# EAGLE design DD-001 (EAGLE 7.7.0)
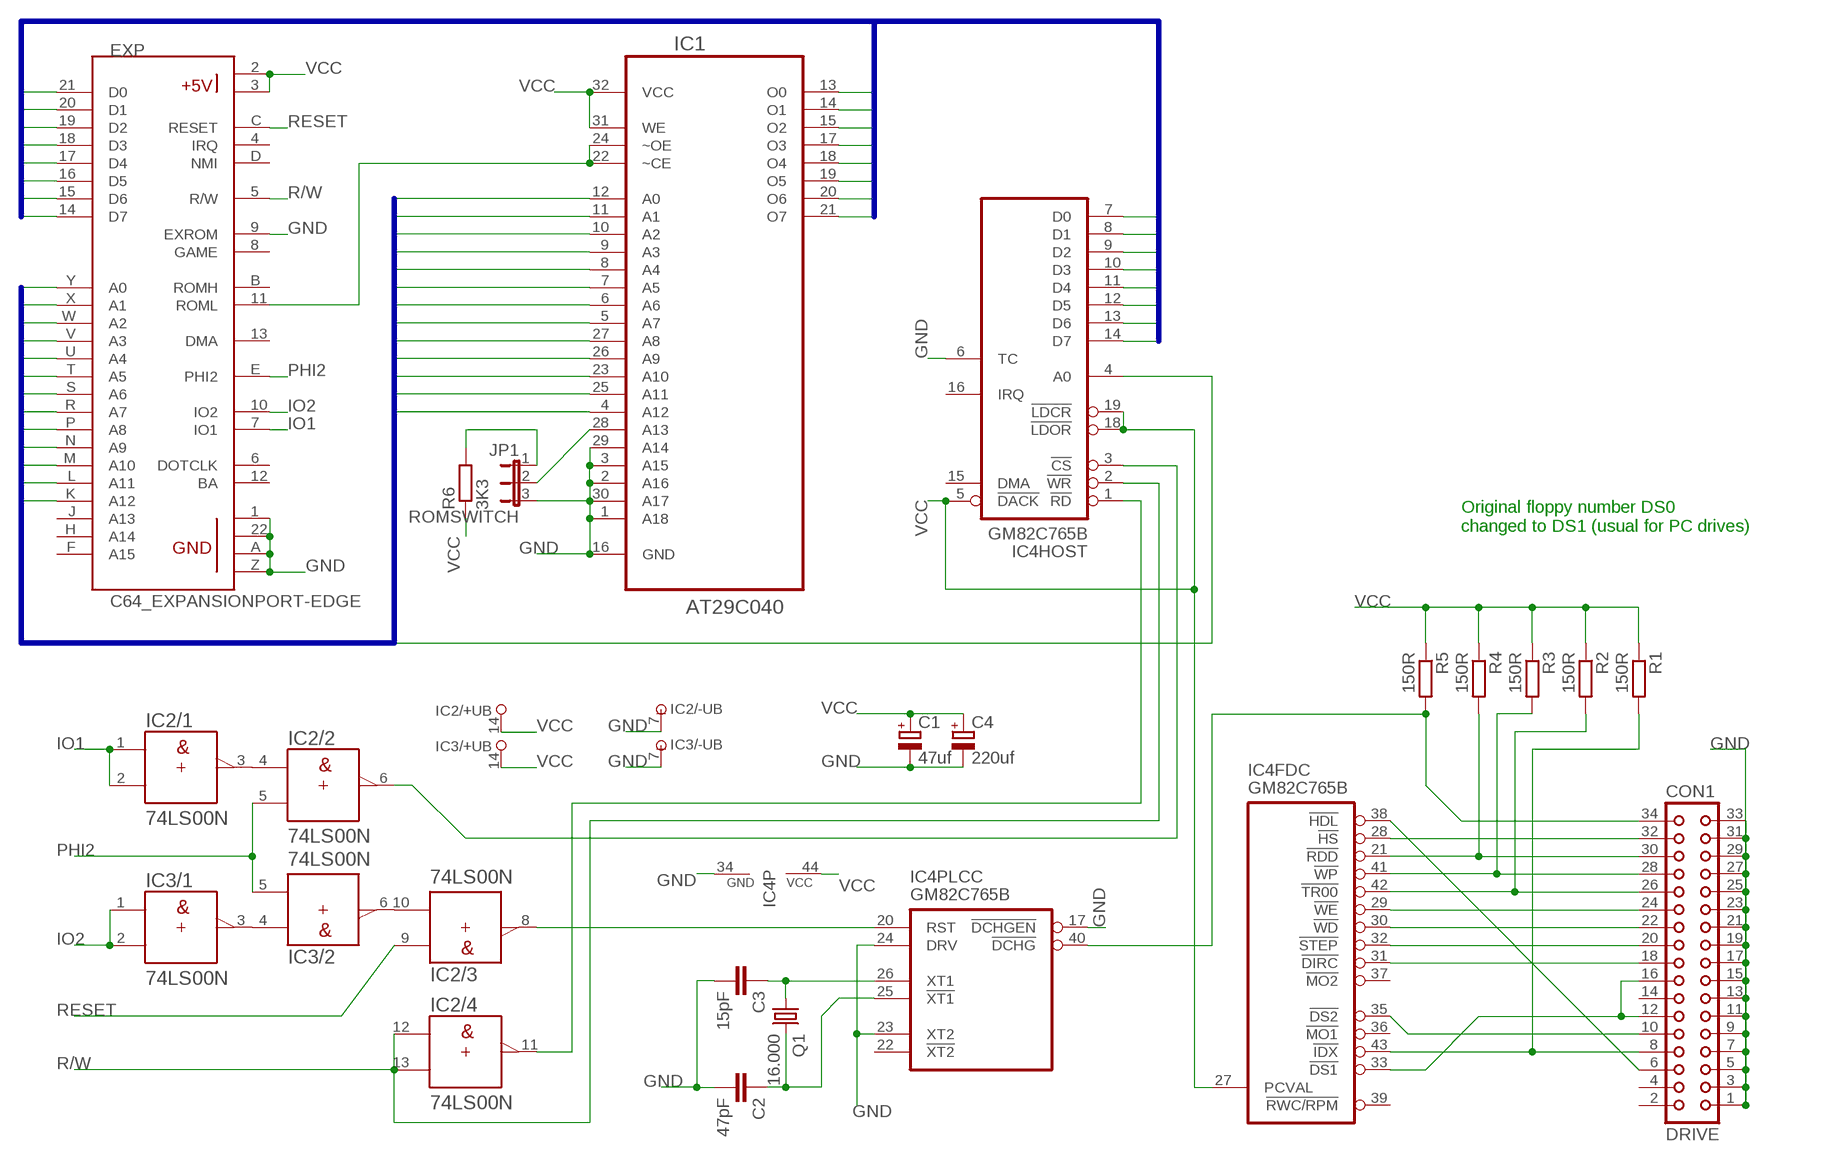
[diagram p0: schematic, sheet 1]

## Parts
C1  47uf  CPOL-EUE2.5-5  [E2,5-5]
C2  47pF  C-EU050-024X044  [C050-024X044]
C3  15pF  C-EU050-024X044  [C050-024X044]
C4  220uf  CPOL-EUE5-6  [E5-6]
CON1  DRIVE  CON34L  [CON34L]
EXP  C64_EXPANSIONPORT-EDGE  [EXPANSIONPORT-C64-EDGE]
IC1  AT29C040  [DIP254P1524X482-32]
IC2  74LS00N  [DIL14]
IC3  74LS00N  [DIL14]
IC4  GM82C765B  3765_PLCC  [PLCC44]
JP1  ROMSWITCH  JP2W  [JP2W]
Q1  16.000  CRYSTALHC49S  [HC49/S]
R1  150R  R-EU_0207/10  [0207/10]
R2  150R  R-EU_0207/10  [0207/10]
R3  150R  R-EU_0207/10  [0207/10]
R4  150R  R-EU_0207/10  [0207/10]
R5  150R  R-EU_0207/10  [0207/10]
R6  3K3  R-EU_R1206  [R1206]

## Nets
_XT1: C2.1 IC4.25(PLCC:!XT1) Q1.2
A0: EXP.Y(A0) IC1.12(A0) IC4.4(HOST:A0)
A1: EXP.X(A1) IC1.11(A1)
A2: EXP.W(A2) IC1.10(A2)
A3: EXP.V(A3) IC1.9(A3)
A4: EXP.U(A4) IC1.8(A4)
A5: EXP.T(A5) IC1.7(A5)
A6: EXP.S(A6) IC1.6(A6)
A7: EXP.R(A7) IC1.5(A7)
A8: EXP.P(A8) IC1.27(A8)
A9: EXP.N(A9) IC1.26(A9)
A10: EXP.M(A10) IC1.23(A10)
A11: EXP.L(A11) IC1.25(A11)
A12: EXP.K(A12) IC1.4(A12)
A13: IC1.28(A13) JP1.2
CS: IC2.6(/2:Y) IC4.3(HOST:!CS)
D0: EXP.21(D0) IC1.13(O0) IC4.7(HOST:D0)
D1: EXP.20(D1) IC1.14(O1) IC4.8(HOST:D1)
D2: EXP.19(D2) IC1.15(O2) IC4.9(HOST:D2)
D3: EXP.18(D3) IC1.17(O3) IC4.10(HOST:D3)
D4: EXP.17(D4) IC1.18(O4) IC4.11(HOST:D4)
D5: EXP.16(D5) IC1.19(O5) IC4.12(HOST:D5)
D6: EXP.15(D6) IC1.20(O6) IC4.13(HOST:D6)
D7: EXP.14(D7) IC1.21(O7) IC4.14(HOST:D7)
DCHG: CON1.34 IC4.40(PLCC:!DCHG) R5.2
DIR: CON1.18 IC4.31(FDC:!DIRC)
DS1: CON1.12 CON1.16 IC4.33(FDC:!DS1)
DS2: CON1.10 IC4.35(FDC:!DS2)
GND: C1.- C2.2 C3.2 C4.- CON1.1 CON1.3 CON1.5 CON1.7 CON1.9 CON1.11 CON1.13 CON1.15 CON1.17 CON1.19 CON1.21 CON1.23 CON1.25 CON1.27 CON1.29 CON1.31 CON1.33 EXP.1(GND1) EXP.9(EXROM) EXP.22(GND2) EXP.A(GND3) EXP.Z(GND4) IC1.1(A18) IC1.2(A16) IC1.3(A15) IC1.16(GND) IC1.29(A14) IC1.30(A17) IC2.7(/-UB:-UB) IC3.7(/-UB:-UB) IC4.6(HOST:TC) IC4.17(PLCC:!DCHGEN) IC4.23(PLCC:XT2) IC4.24(PLCC:DRV) IC4.34(P:GND) JP1.3
HDL: CON1.6 IC4.38(FDC:!HDL)
HI_ROM: JP1.1 R6.2
HS: CON1.32 IC4.28(FDC:!HS)
IDX: CON1.8 IC4.43(FDC:!IDX) R1.2
IO1: EXP.7(IO1) IC2.1(/1:A) IC2.2(/1:B)
IO1N: IC2.3(/1:Y) IC2.4(/2:A)
IO2: EXP.10(IO2) IC3.1(/1:A) IC3.2(/1:B)
IO2N: IC3.3(/1:Y) IC3.4(/2:A)
IO2RES: IC2.10(/3:B) IC3.6(/2:Y)
PHI2: EXP.E(PHI2) IC2.5(/2:B) IC3.5(/2:B)
R/W: EXP.5(R/W) IC2.12(/4:A) IC2.13(/4:B) IC4.2(HOST:!WR)
RD: IC2.11(/4:Y) IC4.1(HOST:!RD)
RDD: CON1.30 IC4.21(FDC:!RDD) R4.2
RESET: EXP.C(RESET) IC2.9(/3:A)
ROML: EXP.11(ROML) IC1.22(~CE) IC1.24(~OE)
RST: IC2.8(/3:Y) IC4.20(PLCC:RST)
STEP: CON1.20 IC4.32(FDC:!STEP)
TR00: CON1.26 IC4.42(FDC:!TR00) R2.2
VCC: C1.+ C4.+ EXP.2(+5V1) EXP.3(+5V2) IC1.31(WE) IC1.32(VCC) IC2.14(/+UB:+UB) IC3.14(/+UB:+UB) IC4.5(HOST:!DACK) IC4.18(HOST:!LDOR) IC4.19(HOST:!LDCR) IC4.27(FDC:PCVAL) IC4.44(P:VCC) R1.1 R2.1 R3.1 R4.1 R5.1 R6.1
WD: CON1.22 IC4.30(FDC:!WD)
WE: CON1.24 IC4.29(FDC:!WE)
WP: CON1.28 IC4.41(FDC:!WP) R3.2
XT1: C3.1 IC4.26(PLCC:XT1) Q1.1
Unconnected: CON1.2 CON1.4 CON1.14 EXP.4(IRQ) EXP.6(DOTCLK) EXP.8(GAME) EXP.12(BA) EXP.13(DMA) EXP.B(ROMH) EXP.D(NMI) EXP.F(A15) EXP.H(A14) EXP.J(A13) IC3.8(/3:Y) IC3.9(/3:A) IC3.10(/3:B) IC3.11(/4:Y) IC3.12(/4:A) IC3.13(/4:B) IC4.15(HOST:DMA) IC4.16(HOST:IRQ) IC4.22(PLCC:!XT2) IC4.36(FDC:!MO1) IC4.37(FDC:!MO2) IC4.39(FDC:!RWC/RPM)

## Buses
D[0..7]
A[0..12]

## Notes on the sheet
- Original floppy number DS0
  changed to DS1 (usual for PC drives)

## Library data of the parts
C1 C4 = resistor:CPOL-EU: POLARIZED CAPACITOR, European symbol
C2 C3 = rcl:C-EU: CAPACITOR, European symbol
CON1 = con-harting:CON34L: CONNECTOR; OC_FARNELL: unknown; OC_NEWARK: unknown
EXP = commodore:C64_EXPANSIONPORT-EDGE: expansion port for the Commodore 64, edge/cartridge version
IC1 = Atmel_By_element14_Batch_1-00:AT29C040: 4-Megabit (512K x 8) OTP EPROM; MPN: AT29C040; OC_FARNELL: 1455024; OC_NEWARK: 58M3822; PACKAGE: PDIP-32; SUPPLIER: Atmel
IC2 IC3 = 74ttl-din:74*00: Quad 2-input NAND gate
IC4 = oldchips3:3765_PLCC: 3765 PLCC Floppy Disk Controller
JP1 = jumper:JP2W: JUMPER
Q1 = crystal:CRYSTAL: CRYSTAL; OC_FARNELL: 1667008; OC_NEWARK: unknown
R1-R6 = resistor:R-EU_: RESISTOR, European symbol

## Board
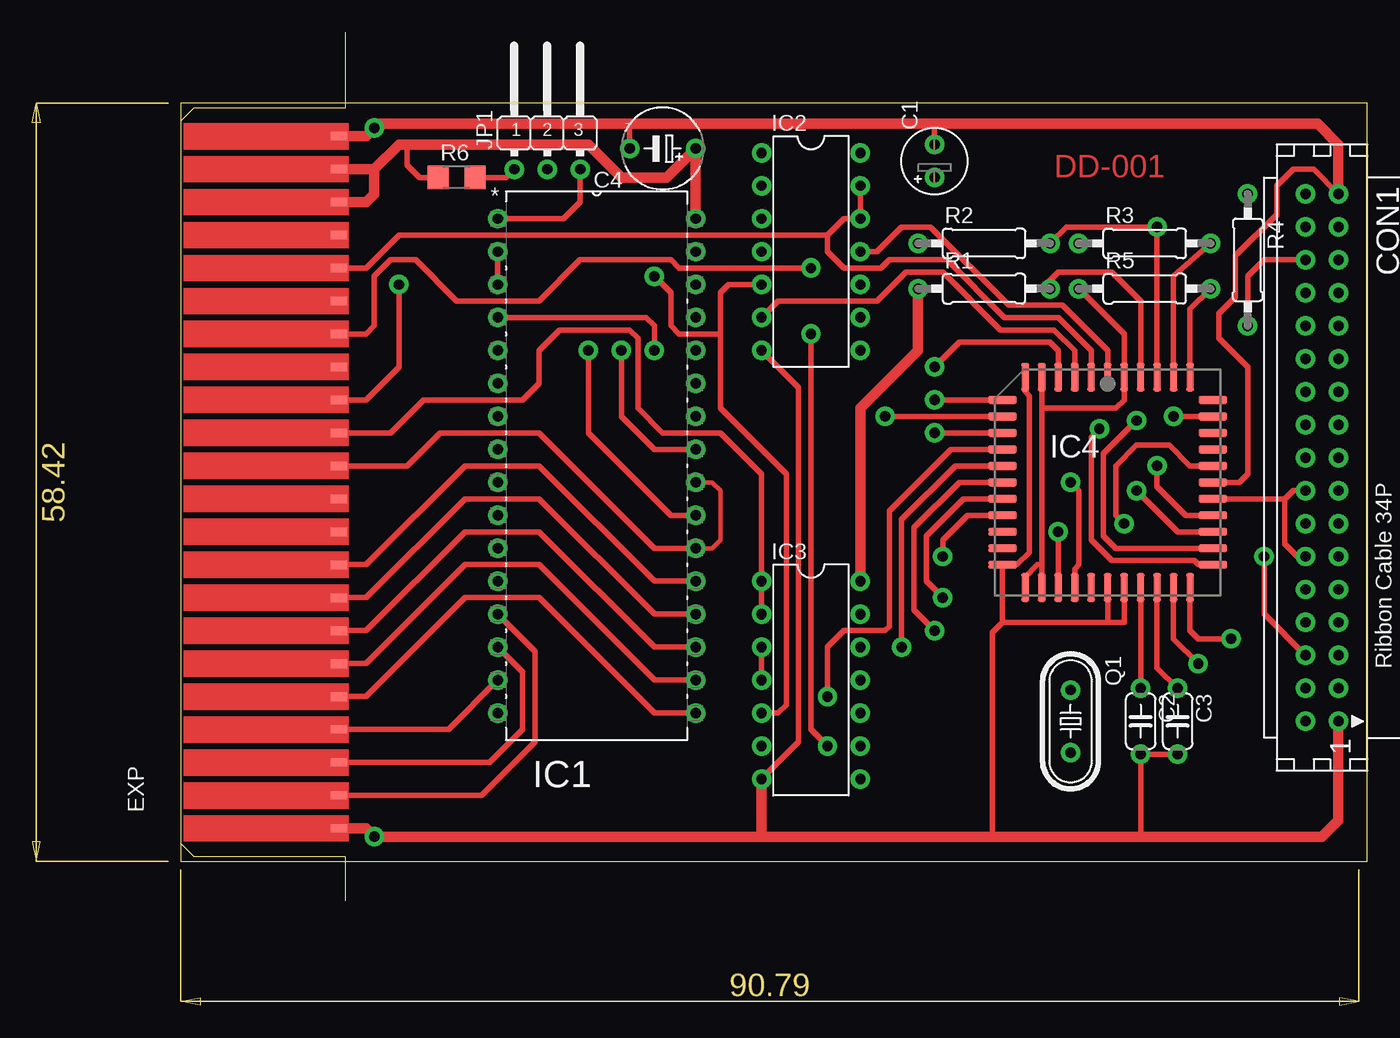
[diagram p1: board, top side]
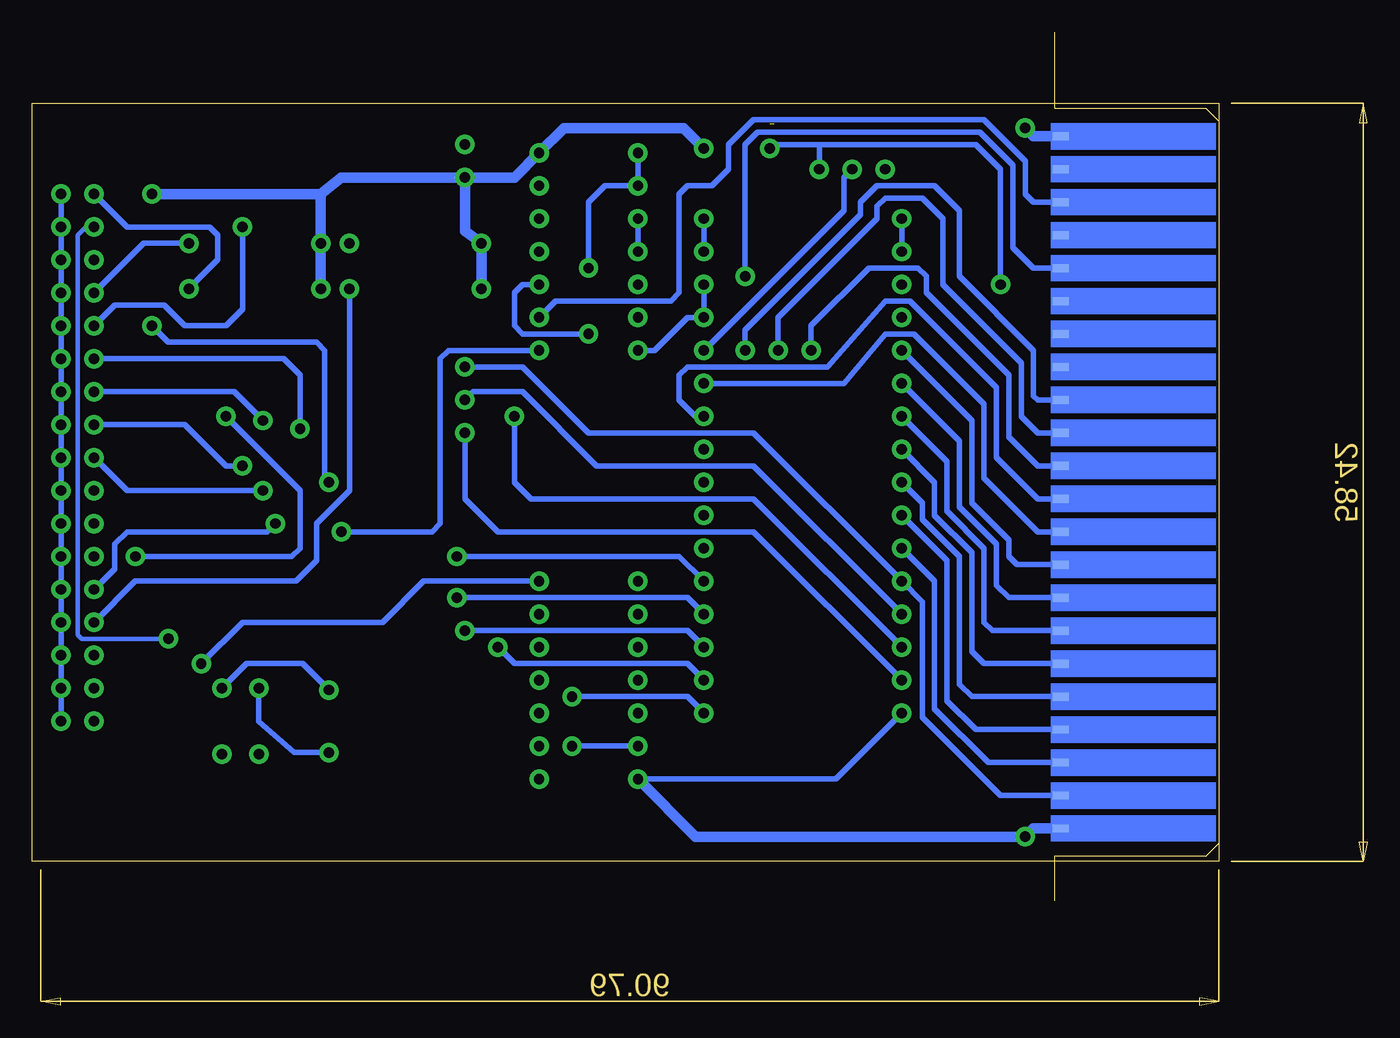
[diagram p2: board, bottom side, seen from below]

Size 102.84 x 74.98 mm. Coordinates in mm from the lower left corner, seen from the top.
Outline: 11.41,11.1 102.84,11.1 102.84,69.5 11.41,69.5 11.41,11.1
Copper layers (1*16): Top 0.035mm / dielectric 1.5mm / Bottom 0.035mm
Design rules "default *": minimum track width 10mil, minimum drill 24mil, track to track 10mil, track to pad 10mil, pad to pad 10mil, via to via 10mil, smd to smd 10mil, copper to edge 40mil, drill to drill 8mil, minimum pad ring 10mil, minimum via ring 8mil, stop-mask expansion 4mil, vias tented up to drill 0mil, thermal gap 10mil

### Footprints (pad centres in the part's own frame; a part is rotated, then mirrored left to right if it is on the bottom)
E2,5-5 = drill 0.8 pad 1.499: + -1.27,0; - 1.27,0
C050-024X044 = drill 0.8 pad 1.499: 1 -2.54,0; 2 2.54,0
E5-6 = drill 0.8 pad 1.499: + -2.54,0; - 2.54,0
CON34L = drill 0.8 pad 1.499: 1 20.32,1.27; 2 20.32,-1.27; 3 17.78,1.27; 4 17.78,-1.27; 5 15.24,1.27; 6 15.24,-1.27; 7 12.7,1.27; 8 12.7,-1.27; 9 10.16,1.27; 10 10.16,-1.27; 11 7.62,1.27; 12 7.62,-1.27; 13 5.08,1.27; 14 5.08,-1.27; 15 2.54,1.27; 16 2.54,-1.27; 17 0,1.27; 18 0,-1.27; 19 -2.54,1.27; 20 -2.54,-1.27; 21 -5.08,1.27; 22 -5.08,-1.27; 23 -7.62,1.27; 24 -7.62,-1.27; 25 -10.16,1.27; 26 -10.16,-1.27; 27 -12.7,1.27; 28 -12.7,-1.27; 29 -15.24,1.27; 30 -15.24,-1.27; 31 -17.78,1.27; 32 -17.78,-1.27; 33 -20.32,1.27; 34 -20.32,-1.27
EXPANSIONPORT-C64-EDGE = smd 0.635 x 1.27: 1 2.54,12.192; 2 5.08,12.192; 3 7.62,12.192; 4 10.16,12.192; 5 12.7,12.192; 6 15.24,12.192; 7 17.78,12.192; 8 20.32,12.192; 9 22.86,12.192; 10 25.4,12.192; 11 27.94,12.192; 12 30.48,12.192; 13 33.02,12.192; 14 35.56,12.192; 15 38.1,12.192; 16 40.64,12.192; 17 43.18,12.192; 18 45.72,12.192; 19 48.26,12.192; 20 50.8,12.192; 21 53.34,12.192; 22 55.88,12.192 | smd 0.635 x 1.27 bottom: A 2.54,12.192; B 5.08,12.192; C 7.62,12.192; D 10.16,12.192; E 12.7,12.192; F 15.24,12.192; H 17.78,12.192; J 20.32,12.192; K 22.86,12.192; L 25.4,12.192; M 27.94,12.192; N 30.48,12.192; P 33.02,12.192; R 35.56,12.192; S 38.1,12.192; T 40.64,12.192; U 43.18,12.192; V 45.72,12.192; W 48.26,12.192; X 50.8,12.192; Y 53.34,12.192; Z 55.88,12.192
DIP254P1524X482-32 = drill 0.8 pad 1.499: 1 -15.24,38.1; 2 -15.24,35.56; 3 -15.24,33.02; 4 -15.24,30.48; 5 -15.24,27.94; 6 -15.24,25.4; 7 -15.24,22.86; 8 -15.24,20.32; 9 -15.24,17.78; 10 -15.24,15.24; 11 -15.24,12.7; 12 -15.24,10.16; 13 -15.24,7.62; 14 -15.24,5.08; 15 -15.24,2.54; 16 -15.24,0; 17 0,0; 18 0,2.54; 19 0,5.08; 20 0,7.62; 21 0,10.16; 22 0,12.7; 23 0,15.24; 24 0,17.78; 25 0,20.32; 26 0,22.86; 27 0,25.4; 28 0,27.94; 29 0,30.48; 30 0,33.02; 31 0,35.56; 32 0,38.1
DIL14 = drill 0.8 pad 1.499: 1 -7.62,-3.81; 2 -5.08,-3.81; 3 -2.54,-3.81; 4 0,-3.81; 5 2.54,-3.81; 6 5.08,-3.81; 7 7.62,-3.81; 8 7.62,3.81; 9 5.08,3.81; 10 2.54,3.81; 11 0,3.81; 12 -2.54,3.81; 13 -5.08,3.81; 14 -7.62,3.81
PLCC44 = smd 0.6 x 2.2: 1 0,6.83; 2 -1.27,6.83; 3 -2.54,6.83; 4 -3.81,6.83; 5 -5.08,6.83; 6 -6.35,6.83; 18 -6.35,-9.37; 19 -5.08,-9.37; 20 -3.81,-9.37; 21 -2.54,-9.37; 22 -1.27,-9.37; 23 0,-9.37; 24 1.27,-9.37; 25 2.54,-9.37; 26 3.81,-9.37; 27 5.08,-9.37; 28 6.35,-9.37; 40 6.35,6.83; 41 5.08,6.83; 42 3.81,6.83; 43 2.54,6.83; 44 1.27,6.83 | smd 2.2 x 0.6: 7 -8.1,5.08; 8 -8.1,3.81; 9 -8.1,2.54; 10 -8.1,1.27; 11 -8.1,0; 12 -8.1,-1.27; 13 -8.1,-2.54; 14 -8.1,-3.81; 15 -8.1,-5.08; 16 -8.1,-6.35; 17 -8.1,-7.62; 29 8.1,-7.62; 30 8.1,-6.35; 31 8.1,-5.08; 32 8.1,-3.81; 33 8.1,-2.54; 34 8.1,-1.27; 35 8.1,0; 36 8.1,1.27; 37 8.1,2.54; 38 8.1,3.81; 39 8.1,5.08
JP2W = drill 0.8 pad 1.499: 1 -2.54,-1.27; 2 0,-1.27; 3 2.54,-1.27
HC49/S = drill 0.8 pad 1.499: 1 -2.413,0; 2 2.413,0
0207/10 = drill 0.8 pad 1.499: 1 -5.08,0; 2 5.08,0
R1206 = smd 1.6 x 1.803: 1 -1.422,0; 2 1.422,0

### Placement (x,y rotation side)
C1  69.52,65.07 90 top
C2  85.39,21.89 270 top
C3  88.25,21.89 270 top
C4  48.56,66.02 180 top
CON1  99.36,42.21 270 top
EXP  11.41,69.52 270 top
IC1  51.1,22.53 0 top
IC2  59.99,58.08 270 top
IC3  59.99,25.07 270 top
IC4  82.85,41.57 0 top
JP1  39.67,65.7 0 top
Q1  79.99,21.89 270 top
R1  73.33,55.23 0 top
R2  73.33,58.72 0 top
R3  85.71,58.72 0 top
R4  93.64,57.45 270 top
R5  85.71,55.23 0 top
R6  32.69,63.8 0 top

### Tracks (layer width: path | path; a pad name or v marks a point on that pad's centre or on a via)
_XT1
  Top 0.406: C2.1 IC4.25
  Bottom 0.406: Q1.2 82.66,19.48 85.39,21.89 C2.1
A0  (via drill 0.8 pad 1.5)
  Top 0.406: v69.52,49.2 71.42,51.1 78.41,51.1 79.04,50.46 IC4.4
  Bottom 0.406: v69.52,49.2 65.07,49.2 59.99,44.11 47.29,44.11 IC1.12 34.27,31.1 34.27,22.21 28.24,16.18 EXP.Y
A1
  Bottom 0.406: IC1.11 33.32,32.68 33.32,22.84 29.19,18.71 EXP.X
A2
  Bottom 0.406: IC1.10 32.37,34.27 32.37,23.48 30.15,21.26 EXP.W
A3
  Bottom 0.406: IC1.9 34.27,38.72 34.27,37.45 31.41,34.59 31.41,24.75 30.46,23.8 EXP.V
A4
  Bottom 0.406: IC1.8 33.32,40.3 33.32,37.77 30.46,34.91 30.46,27.29 29.51,26.34 EXP.U
A5
  Bottom 0.406: IC1.7 32.37,41.89 32.37,38.08 29.51,35.22 29.51,29.51 28.88,28.88 EXP.T
A6
  Bottom 0.406: IC1.6 31.41,43.48 31.41,38.4 28.56,35.54 28.56,32.37 27.61,31.42 EXP.S
A7
  Bottom 0.406: IC1.5 30.46,45.07 30.46,38.72 27.61,35.86 27.61,34.59 26.97,33.95 EXP.R
A8
  Bottom 0.406: IC1.27 40.3,47.92 37.13,51.73 34.91,51.73 29.51,46.34 29.51,40.62 25.38,36.49 EXP.P
A9
  Bottom 0.406: IC1.26 51.73,45.38 53.01,46.66 53.01,48.56 52.37,49.2 41.58,49.2 37.13,54.27 35.23,54.27 28.56,47.61 28.56,42.21 25.38,39.03 EXP.N 23.8,39.03
A10  (via drill 0.8 pad 1.5)
  Top 0.406: v42.85,50.46 42.85,44.11 49.2,37.77 IC1.23
  Bottom 0.406: v42.85,50.46 42.85,52.37 38.4,56.81 34.59,56.81 33.95,56.18 33.95,54.91 27.61,48.56 27.61,43.8 25.38,41.57 EXP.M
A11  (via drill 0.8 pad 1.5)
  Top 0.406: v45.39,50.46 45.39,45.38 47.93,42.84 IC1.25
  Bottom 0.406: v45.39,50.46 45.39,53 37.77,60.62 37.77,61.58 37.13,62.21 34.27,62.21 32.69,60.62 32.69,55.54 26.65,49.51 26.65,45.38 25.38,44.11 EXP.L
A12  (via drill 0.8 pad 1.5)
  Top 0.406: IC1.4 47.29,53 47.93,52.37 v47.93,50.46
  Bottom 0.406: v47.93,50.46 47.93,52.05 39.04,60.94 39.04,61.89 37.77,63.16 33.32,63.16 31.41,61.26 31.41,56.18 25.7,50.46 25.7,46.97 25.38,46.66 EXP.K
A13
  Bottom 0.406: IC1.28 40.3,61.26 40.3,63.8 JP1.2
CS
  Top 0.406: IC4.3 80.31,50.46 78.72,52.05 74.59,52.05 70.15,56.5 67.29,56.5 65.07,54.27 57.45,54.27 IC2.6
D0  (via drill 0.8 pad 1.5)
  Top 0.406: IC1.13 38.72,27.29 38.72,20.3 34.59,16.18 EXP.21 | IC4.7 v69.52,46.66
  Bottom 0.406: v69.52,46.66 68.88,47.29 65.07,47.29 59.36,41.57 47.29,41.57 IC1.13
D1  (via drill 0.8 pad 1.5)
  Top 0.406: IC1.14 37.77,25.7 37.77,21.26 35.23,18.71 EXP.20 | IC4.8 v65.7,45.38
  Bottom 0.406: IC1.14 47.29,39.03 64.44,39.03 65.7,40.3 v65.7,45.38
D2  (via drill 0.8 pad 1.5)
  Top 0.406: IC1.15 32.05,21.26 EXP.19 23.8,21.26 | IC4.9 v69.52,44.11
  Bottom 0.406: IC1.15 47.29,36.49 66.97,36.49 69.52,39.03 v69.52,44.11
D3  (via drill 0.8 pad 1.5)
  Top 0.406: EXP.18 25.7,23.8 33.32,31.42 39.04,31.42 47.93,22.53 IC1.17 | v61.26,23.8 61.26,27.61 62.53,28.88 65.7,28.88 66.02,29.19 66.02,38.08 70.78,42.84 IC4.10
  Bottom 0.406: v61.26,23.8 52.37,23.8 IC1.17
D4  (via drill 0.8 pad 1.5)
  Top 0.406: EXP.17 25.7,26.34 33.32,33.95 39.04,33.95 47.93,25.07 IC1.18 | v66.97,27.61 66.97,37.45 71.1,41.57 IC4.11
  Bottom 0.406: v66.97,27.61 65.7,26.34 52.37,26.34 IC1.18
D5  (via drill 0.8 pad 1.5)
  Top 0.406: EXP.16 25.7,28.88 33.32,36.49 39.04,36.49 47.93,27.61 IC1.19 | v69.52,28.88 67.93,30.46 67.93,36.81 71.42,40.3 IC4.12
  Bottom 0.406: v69.52,28.88 52.37,28.88 IC1.19
D6  (via drill 0.8 pad 1.5)
  Top 0.406: EXP.15 25.7,31.42 33.32,39.03 39.04,39.03 47.93,30.14 IC1.20 | v70.15,31.42 68.88,32.68 68.88,36.18 71.74,39.03 IC4.13
  Bottom 0.406: IC1.20 52.37,31.42 v70.15,31.42
D7  (via drill 0.8 pad 1.5)
  Top 0.406: EXP.14 25.7,33.95 33.32,41.57 39.04,41.57 47.93,32.68 IC1.21 | v70.15,34.59 70.15,35.86 72.05,37.77 IC4.14
  Bottom 0.406: v70.15,34.59 53.01,34.59 IC1.21
DCHG
  Top 0.406: IC4.40 89.2,53.64 R5.2
  Bottom 0.406: R5.2 88.56,57.45 88.56,59.36 89.2,59.99 95.55,59.99 CON1.34
DIR  (via drill 0.8 pad 1.5)
  Top 0.406: v85.07,39.67 88.25,36.49 IC4.31
  Bottom 0.406: CON1.18 95.55,39.67 v85.07,39.67
DS1
  Top 0.406: CON1.12 97.45,34.59 96.5,35.54 96.5,39.03 | 96.5,39.03 97.14,39.67 CON1.16 | IC4.33 96.5,39.03
DS2  (via drill 0.8 pad 1.5)
  Top 0.406: IC4.35 89.2,41.57 87.61,43.16 85.07,43.16 83.48,41.57 83.48,37.77 v84.12,37.13
  Bottom 0.406: CON1.10 96.5,33.64 96.5,35.54 95.55,36.49 84.76,36.49 v84.12,37.13
GND  (via drill 0.8 pad 1.5)  (1 unrouted)
  Top 0.406: v28.24,55.54 28.24,49.2 25.7,46.66 EXP.9 | EXP.Z 23.8,13.64 | IC2.7 59.04,47.61 59.04,20.3 IC3.7 | IC1.3 IC1.2 | IC1.1 40.94,60.62 42.21,61.89 JP1.3 | 46.02,67.93 C4.- | 23.8,66.97 EXP.A | C3.2 C2.2 85.39,13 | 74.75,29.51 IC4.17 75.87,33.95 76.82,34.91 76.82,46.97 76.5,47.29 IC4.6 | 82.85,29.51 84.12,29.51 IC4.24 | 82.85,29.51 74.75,29.51 | IC4.34 93.01,40.3 93.64,40.94 93.64,49.2 91.42,51.42 91.42,53.32 92.69,54.59 92.69,57.77 95.87,60.94 95.87,63.16 97.14,64.44 98.73,64.44 CON1.33 | C1.- 69.52,67.93 | v26.34,67.61 26.65,67.93 | 74.75,29.51 73.96,28.72 73.96,13 | IC4.23 82.85,29.51
  Top 0.813: 56.18,13 v26.34,13 25.7,13.64 EXP.Z | 56.18,13 IC3.7 | CON1.1 100.63,14.27 99.36,13 85.39,13 73.96,13 56.18,13 | CON1.33 100.63,66.34 99.04,67.93 69.52,67.93 46.02,67.93 | EXP.A 25.7,66.97 v26.34,67.61 | 26.65,67.93 45.7,67.93
  Bottom 0.406: v28.24,55.54 28.24,64.44 30.15,66.34 42.21,66.34 | EXP.Z 23.8,13.64 | IC3.7 40.94,17.45 IC1.16 | IC1.30 IC1.29 52.37,53 54.91,50.46 IC2.7 | JP1.3 42.21,66.34 | IC1.2 IC1.1 | EXP.A 23.8,66.97 | CON1.33 CON1.31 CON1.29 CON1.27 CON1.25 CON1.23 CON1.21 CON1.19 CON1.17 CON1.15 CON1.13 CON1.11 CON1.9 CON1.7 CON1.5 CON1.3 CON1.1 | C4.- 45.7,66.34 42.21,66.34
  Bottom 0.813: IC3.7 51.73,13 v26.34,13 25.7,13.64 EXP.Z | EXP.A 25.7,66.97 v26.34,67.61
HDL  (via drill 0.8 pad 1.5)
  Top 0.406: IC4.38 v87.93,45.38 | CON1.6 94.92,30.14 v94.92,34.59
  Bottom 0.406: v94.92,34.59 82.85,34.59 82.22,35.22 82.22,39.67 v87.93,45.38
HI_ROM
  Top 0.406: JP1.1 36.5,63.8 R6.2
HS  (via drill 0.8 pad 1.5)
  Top 0.406: IC4.28 89.2,28.88 89.84,28.24 v92.38,28.24
  Bottom 0.356: v92.38,28.24 99.04,28.24 99.36,28.56 99.36,58.72 99.36,59.36 98.73,59.99 CON1.32
IDX
  Top 0.406: IC4.43 85.39,54.27 83.17,56.5 79.04,56.5 78.41,55.86 R1.2
  Bottom 0.406: CON1.8 94.92,32.68 82.53,32.68 80.95,34.27 80.95,37.13 78.41,39.67 R1.2
IO1  (via drill 0.8 pad 1.5)
  Top 0.406: EXP.7 25.7,51.73 26.34,52.37 26.34,56.18 27.61,57.45 29.51,57.45 32.69,54.27 39.04,54.27 42.21,57.45 49.2,57.45 49.83,56.81 v59.99,56.81
  Bottom 0.406: v59.99,56.81 59.99,61.89 58.72,63.16 IC2.2 IC2.1
IO1N
  Bottom 0.406: IC2.3 IC2.4
IO2
  Top 0.406: EXP.10 27.61,44.11 30.15,46.66 37.77,46.66 39.04,47.92 39.04,50.46 40.62,52.05 46.02,52.05 46.66,51.42 46.66,46.02 48.56,44.11 53.01,44.11 56.18,40.94 IC3.1 IC3.2
IO2N
  Top 0.406: IC3.4 IC3.3
IO2RES  (via drill 0.8 pad 1.5)
  Top 0.406: v59.99,51.73 59.99,21.26 v61.26,19.99
  Bottom 0.406: IC2.10 65.07,55.54 65.7,54.91 65.7,52.37 65.07,51.73 v59.99,51.73 | v61.26,19.99 IC3.6
PHI2  (via drill 0.8 pad 1.5)
  Top 0.406: IC2.5 53.64,55.54 53.01,54.91 53.01,51.73 | v47.93,56.18 49.2,54.91 49.2,52.37 49.83,51.73 53.01,51.73 | 53.01,51.73 53.01,46.02 58.09,40.94 58.09,23.16 57.45,22.53 IC3.5
  Bottom 0.406: v47.93,56.18 47.93,66.34 46.97,67.29 29.83,67.29 27.29,64.75 27.29,58.4 25.7,56.81 EXP.E
R/W
  Top 0.406: EXP.5 25.7,56.81 28.24,59.36 61.26,59.36 | IC2.13 IC2.12 62.53,60.62 61.26,59.36 | 61.26,59.36 61.26,58.08 62.53,56.81 65.39,56.81 66.02,57.45 70.47,57.45 74.91,53 79.04,53 81.58,50.46 IC4.2
RD
  Top 0.406: IC4.1 82.85,50.46 79.36,53.96 75.23,53.96 69.2,59.99 66.97,59.99 65.07,58.08 IC2.11
RDD  (via drill 0.8 pad 1.5)
  Top 0.406: R4.2 93.64,56.18 94.92,57.45 CON1.30 | v79.99,40.3 80.63,39.67 80.63,33.95 80.31,33.64 IC4.21
  Bottom 0.406: R4.2 92.38,51.1 80.95,51.1 80.31,50.46 80.31,40.62 v79.99,40.3
RESET
  Bottom 0.406: 25.07,61.89 EXP.C 25.7,61.89 26.34,62.53 26.34,65.07 29.51,68.25 47.29,68.25 49.2,66.34 49.2,64.44 50.47,63.16 52.37,63.16 53.01,62.53 53.01,54.91 53.64,54.27 62.53,54.27 IC2.9
ROML
  Top 0.356: IC1.22 52.37,35.22 53.01,35.86 53.01,39.67 52.37,40.3 IC1.24
  Top 0.406: EXP.11 28.88,41.57 31.41,44.11 39.04,44.11 47.93,35.22 IC1.22
RST  (via drill 0.8 pad 1.5)
  Top 0.406: v79.04,36.49 IC4.20
  Bottom 0.406: v79.04,36.49 72.05,36.49 71.42,37.13 71.42,49.83 70.78,50.46 IC2.8
STEP  (via drill 0.8 pad 1.5)
  Top 0.406: v86.66,41.57 86.66,39.99 88.88,37.77 IC4.32
  Bottom 0.406: CON1.20 91.11,44.75 87.93,41.57 v86.66,41.57
TR00  (via drill 0.8 pad 1.5)
  Top 0.406: IC4.42 v86.66,59.99 79.67,59.99 R2.2
  Bottom 0.406: v86.66,59.99 86.66,53.64 87.93,52.37 91.11,52.37 92.69,53.96 96.5,53.96 CON1.26
VCC  (via drill 0.8 pad 1.5)
  Top 0.406: R5.1 84.12,51.73 IC4.44 84.12,46.66 83.48,46.02 77.77,46.02 | 77.77,33.95 77.77,46.02 | v89.84,26.34 87.93,28.24 IC4.27 | 77.77,33.95 77.45,33.95 76.5,33 IC4.18 | IC4.19 77.77,33.95 | 77.77,46.02 IC4.5 | R6.1 29.83,63.8 28.88,64.75 28.88,66.34
  Top 0.813: 26.34,64.44 28.24,66.34 28.88,66.34 42.85,66.34 45.39,63.8 48.88,63.8 C4.+ IC1.32 | EXP.2 26.34,64.44 | 26.34,64.44 26.34,62.53 25.7,61.89 EXP.3 | R1.1 68.25,50.46 63.8,46.02 IC3.14
  Bottom 0.406: IC1.32 IC1.31 | v89.84,26.34 86.66,29.51 75.87,29.51 72.69,32.68 IC3.14
  Bottom 0.813: R1.1 R2.1 69.52,59.67 C1.+ | R5.1 R3.1 80.63,62.53 | 80.63,62.53 79.04,63.8 C1.+ | C4.+ 52.69,67.61 61.9,67.61 IC2.14 65.7,63.8 C1.+ | R4.1 80.63,62.53
WD  (via drill 0.8 pad 1.5)
  Top 0.406: IC4.30 83.48,35.22 82.53,36.18 82.53,41.57 82.53,41.89 82.53,42.53 v85.07,45.07
  Bottom 0.406: CON1.22 87.3,47.29 v85.07,45.07
WE  (via drill 0.8 pad 1.5)
  Top 0.406: v82.22,44.43 81.58,43.8 81.58,35.86 83.17,34.27 89.52,34.27 89.84,33.95 IC4.29
  Bottom 0.406: CON1.24 83.48,49.83 82.22,48.56 v82.22,44.43
WP
  Top 0.406: R3.2 87.93,56.18 IC4.41
  Bottom 0.406: R3.2 94.28,58.72 CON1.28
XT1
  Top 0.406: C3.1 86.66,26.02 IC4.26
  Bottom 0.406: Q1.1 82.03,26.34 86.34,26.34 C3.1

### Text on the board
Top: DD-001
